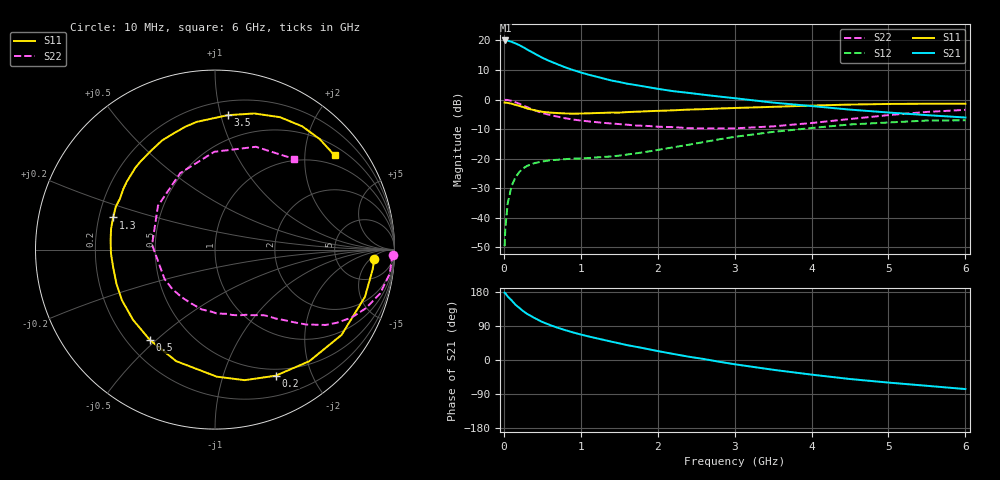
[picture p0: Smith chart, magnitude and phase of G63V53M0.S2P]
! SIEMENS Small Signal Semiconductors
! BFG193
! Si NPN RF Bipolar Junction Transistor in SOT223
! VCE = 3.5 V  IC = 3 mA
! Common Emitter S-Parameters:  August  1996
# GHz  S  MA  R  50
!  f  S11  S21  S12  S22
! GHz  MAG  ANG  MAG  ANG  MAG  ANG  MAG  ANG
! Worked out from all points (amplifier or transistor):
!   36 points, 10 MHz to 6 GHz, reference 50 ohm
!   highest |S21| = 20.0 dB at 20 MHz (marker M1)
!   |S21| within 3 dB of that: start of sweep to 298.6 MHz
!   unconditionally stable (mu >= 1): 1.283 GHz to 2.575 GHz
!   at 250 MHz: K = 0.23, MSG = 20.5 dB, |S12| = -23.3 dB
!   at 1.4 GHz: K = 1.06, MAG = 11.3 dB, |S12| = -19.3 dB
!   at 6 GHz: K = 0.92, MSG = 0.5 dB, |S12| = -7.0 dB
!   S11 on the Smith chart (normalised r, x): 10 MHz: 13, -7; 200 MHz: 0.42, -1.51; 500 MHz: 0.29, -0.48; 1.3 GHz: 0.26, +0.14; 3.5 GHz: 0.30, +1.05; 6 GHz: 0.73, +2.72
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0.01  0.8894 -3.5  9.963 177.5  0.0033 92.5  0.9943 -1.6
0.02  0.8851 -7.2  9.99 176.0  0.0067 87.2  0.9862 -3.1
0.05  0.8761 -17.5  9.901 167.5  0.0175 80.2  0.9832 -7.8
0.1  0.8504 -34.0  9.505 157.7  0.0342 72.8  0.9521 -14.9
0.15  0.8141 -49.8  8.913 146.1  0.0479 63.4  0.9013 -21.3
0.2  0.7797 -64.3  8.347 137.7  0.0592 57.0  0.8502 -26.4
0.25  0.746 -77.2  7.691 129.2  0.0682 51.2  0.7918 -31.0
0.3  0.708 -89.2  7.055 122.1  0.0752 46.8  0.745 -34.3
0.4  0.658 -109.2  5.991 110.7  0.084 39.5  0.6559 -39.5
0.5  0.6203 -125.9  5.093 100.3  0.0894 34.3  0.5913 -43.0
0.6  0.6014 -139.4  4.448 92.3  0.0937 31.0  0.547 -45.8
0.7  0.5903 -151.3  3.934 85.1  0.0958 29.2  0.5122 -48.6
0.9  0.5759 -170.0  3.155 72.7  0.1 27.6  0.4584 -53.0
1.1  0.5837 175.1  2.636 62.3  0.1023 27.6  0.4266 -58.9
1.3  0.5949 162.5  2.264 53.0  0.107 28.9  0.402 -64.6
1.6  0.6125 146.5  1.856 39.3  0.1171 31.2  0.3758 -75.6
2.2  0.6564 122.7  1.387 16.1  0.1553 33.0  0.3414 -102.5
2.8  0.7046 103.5  1.124 -4.6  0.2123 27.5  0.3238 -137.3
3.5  0.7523 84.6  0.887 -25.8  0.2833 13.3  0.3516 175.6
4.5  0.8217 63.9  0.675 -50.2  0.3784 -9.0  0.468 114.5
5.5  0.8482 46.6  0.544 -68.1  0.4411 -36.6  0.6166 68.3
6  0.8483 38.2  0.496 -76.7  0.4449 -51.8  0.6691 49.1
